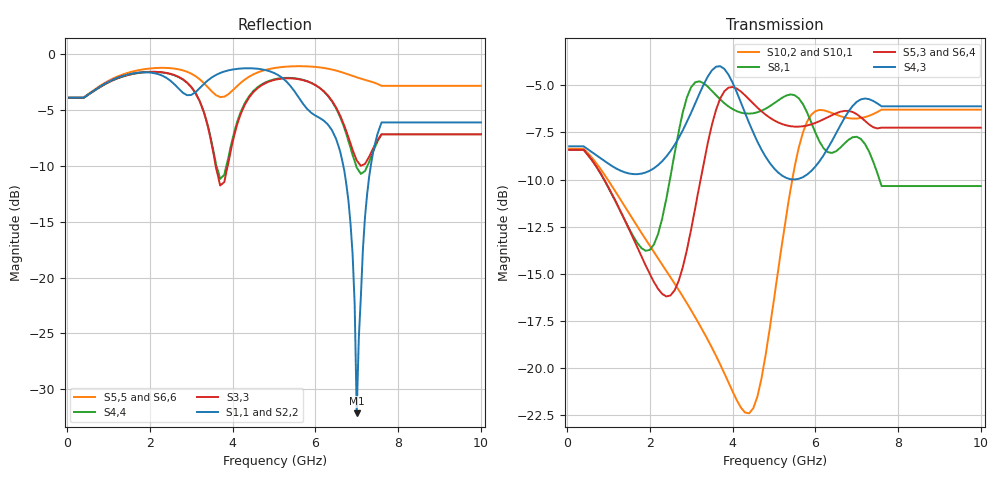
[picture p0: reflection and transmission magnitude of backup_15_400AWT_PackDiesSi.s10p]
! Created Sun Apr 17 16:15:49 2016
# ghz S ma R 50
! 10 Port Network Data from SP1.SP block
! freq  magS1_1  angS1_1  magS1_2  angS1_2  magS1_3  angS1_3  magS1_4  angS1_4
!  magS1_5  angS1_5  magS1_6  angS1_6  magS1_7  angS1_7  magS1_8  angS1_8
!  magS1_9  angS1_9  magS1_10  angS1_10
!  magS2_1  angS2_1  magS2_2  angS2_2
!  magS2_3  angS2_3  magS2_4  angS2_4  magS2_5  angS2_5  magS2_6  angS2_6
!  magS2_7  angS2_7  magS2_8  angS2_8  magS2_9  angS2_9  magS2_10  angS2_10
!  magS3_1  angS3_1  magS3_2  angS3_2  magS3_3  angS3_3  magS3_4  angS3_4
!  magS3_5  angS3_5  magS3_6  angS3_6  magS3_7  angS3_7  magS3_8  angS3_8
!  magS3_9  angS3_9  magS3_10  angS3_10
!  magS4_1  angS4_1  magS4_2  angS4_2
!  magS4_3  angS4_3  magS4_4  angS4_4  magS4_5  angS4_5  magS4_6  angS4_6
!  magS4_7  angS4_7  magS4_8  angS4_8  magS4_9  angS4_9  magS4_10  angS4_10
!  magS5_1  angS5_1  magS5_2  angS5_2  magS5_3  angS5_3  magS5_4  angS5_4
!  magS5_5  angS5_5  magS5_6  angS5_6  magS5_7  angS5_7  magS5_8  angS5_8
!  magS5_9  angS5_9  magS5_10  angS5_10
!  magS6_1  angS6_1  magS6_2  angS6_2
!  magS6_3  angS6_3  magS6_4  angS6_4  magS6_5  angS6_5  magS6_6  angS6_6
!  magS6_7  angS6_7  magS6_8  angS6_8  magS6_9  angS6_9  magS6_10  angS6_10
!  magS7_1  angS7_1  magS7_2  angS7_2  magS7_3  angS7_3  magS7_4  angS7_4
!  magS7_5  angS7_5  magS7_6  angS7_6  magS7_7  angS7_7  magS7_8  angS7_8
!  magS7_9  angS7_9  magS7_10  angS7_10
!  magS8_1  angS8_1  magS8_2  angS8_2
!  magS8_3  angS8_3  magS8_4  angS8_4  magS8_5  angS8_5  magS8_6  angS8_6
!  magS8_7  angS8_7  magS8_8  angS8_8  magS8_9  angS8_9  magS8_10  angS8_10
!  magS9_1  angS9_1  magS9_2  angS9_2  magS9_3  angS9_3  magS9_4  angS9_4
!  magS9_5  angS9_5  magS9_6  angS9_6  magS9_7  angS9_7  magS9_8  angS9_8
!  magS9_9  angS9_9  magS9_10  angS9_10
!  magS10_1  angS10_1  magS10_2  angS10_2
!  magS10_3  angS10_3  magS10_4  angS10_4  magS10_5  angS10_5  magS10_6  angS10_6
!  magS10_7  angS10_7  magS10_8  angS10_8  magS10_9  angS10_9  magS10_10  angS10_10
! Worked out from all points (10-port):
!   200 points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, 50 MHz to 10 GHz, reference 50 ohm
!   strongest paths, dB at 50 MHz, 2.55 GHz, 5.05 GHz, 7.55 GHz, 10 GHz:
!     S4,3: -8.2, -8.3, -9.5, -6.0, -6.1
!     S5,3: -8.4, -16.0, -6.9, -7.3, -7.2
!     S6,4: -8.4, -15.9, -7.1, -7.5, -7.5
!     S8,1: -8.4, -9.2, -5.9, -10.0, -10.3
!     S10,2: -8.4, -15.4, -15.6, -6.4, -6.3
!     S10,1: -8.4, -15.4, -15.9, -6.7, -6.6
!   lowest |S11| = -32.1 dB at 7 GHz (marker M1), VSWR 1.05, Z = 49.2 + j2.32 ohm
!   |S11| at or under -10 dB: 6.676 GHz to 7.34 GHz (663.1 MHz wide, 9.46 % of centre)
